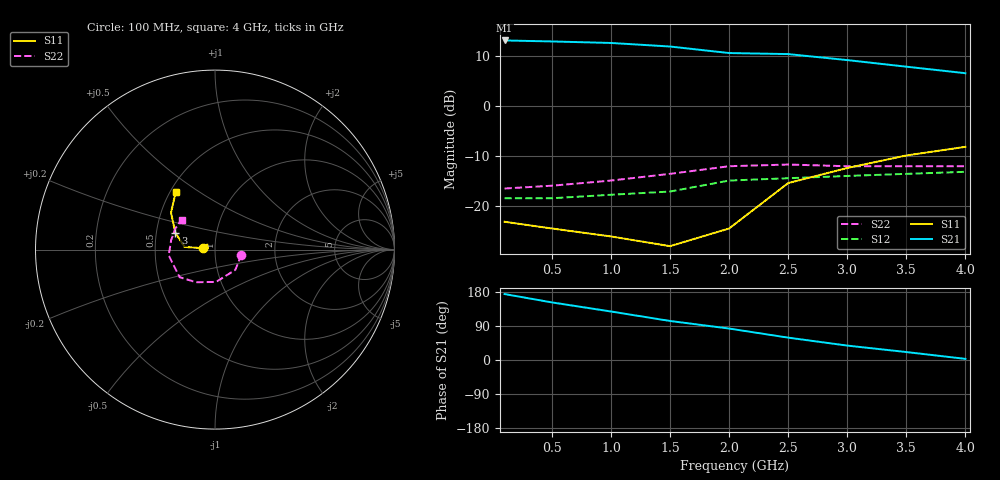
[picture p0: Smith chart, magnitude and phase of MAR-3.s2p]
! MAR-3.535  Mini Circuits
! MAR-3
! V=5V; I=35mA
! S-PARAMETER DATA
#  MHz  S  MA  R  50
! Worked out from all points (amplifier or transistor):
!   9 points, 100 MHz to 4 GHz, reference 50 ohm
!   highest |S21| = 13.0 dB at 100 MHz (marker M1)
!   |S21| within 3 dB of that: start of sweep to 2.619 GHz
!   unconditionally stable (mu >= 1): start of sweep to end of sweep
!   at 500 MHz: K = 1.18, MAG = 13.0 dB, |S12| = -18.4 dB
!   at 2 GHz: K = 1.07, MAG = 11.1 dB, |S12| = -14.9 dB
!   at 4 GHz: K = 1.08, MAG = 8.1 dB, |S12| = -13.2 dB
!   S11 on the Smith chart (normalised r, x): 100 MHz: 0.87, +0.02; 3 GHz: 0.63, +0.13; 4 GHz: 0.53, +0.41
100  0.07 172.0  4.47 174.0  0.12 1.0  0.15 -11.0
500  0.06 156.0  4.37 152.0  0.12 5.0  0.16 -45.0
1000  0.05 146.0  4.22 128.0  0.13 10.0  0.18 -88.0
1500  0.04 172.0  3.89 103.0  0.14 12.0  0.21 -120.0
2000  0.06 173.0  3.35 83.0  0.18 11.0  0.25 -142.0
2500  0.17 175.0  3.27 59.0  0.19 5.0  0.26 -173.0
3000  0.24 157.0  2.85 38.0  0.2 -0.0  0.25 168.0
3500  0.32 140.0  2.45 21.0  0.21 -6.0  0.25 152.0
4000  0.39 124.0  2.11 3.0  0.22 -14.0  0.25 138.0
